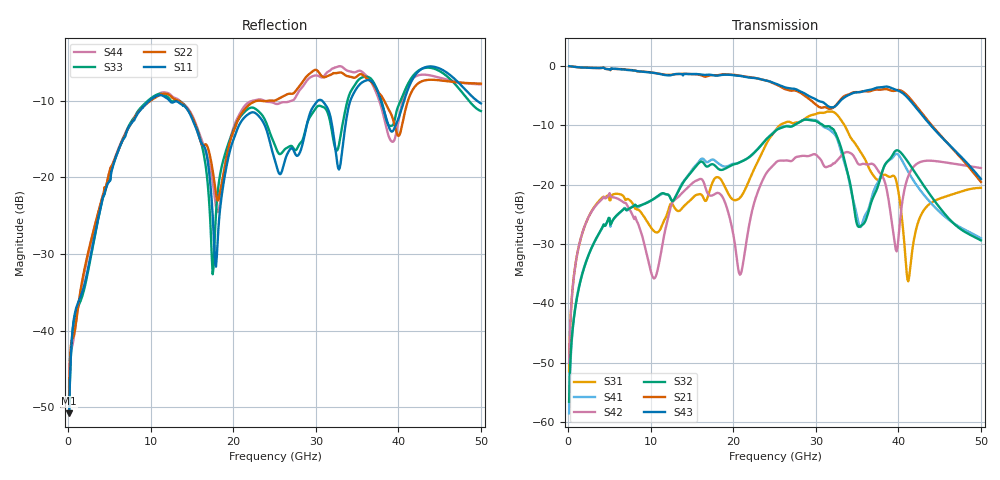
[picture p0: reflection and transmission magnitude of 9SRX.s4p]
! DAC39RF10ACK
! 256-pin FCBGA package
! Texas Instruments 8/20/2022
! Single-ended  S-parameters
! PORT#  PORT_NAME  NET_NAME
! PORT1:  xSRXN.DIEBUMP  xSRXN
! PORT2:  xSRXN.BGA  xSRXN
! PORT3:  xSRXP.DIEBUMP  xSRXP
! PORT4:  xSRXP.BGA  xSRXP
! Touchstone Ver. 1.0
! Number of ports is 4
# Hz	S	MA	R	50.000000
! SCATTERING PARAMETERS  :
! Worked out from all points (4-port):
!   500 points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, 100 MHz to 50 GHz, reference 50 ohm
!   strongest paths, dB at 100 MHz, 12.6 GHz, 25.1 GHz, 37.6 GHz, 50 GHz:
!     S43: 0.0, -1.5, -3.0, -3.6, -19.0
!     S21: 0.0, -1.4, -3.1, -4.0, -19.5
!     S32: -56.5, -22.8, -10.9, -19.9, -29.4
!     S42: -50.0, -23.0, -16.3, -17.7, -17.2
!     S41: -58.5, -22.7, -10.9, -19.4, -29.0
!     S31: -51.4, -23.2, -10.8, -19.2, -20.5
!   lowest |S11| = -50.8 dB at 100 MHz (marker M1), VSWR 1.01, Z = 50.3 + j0.118 ohm
!   |S11| at or under -10 dB: start of sweep to 9.858 GHz; 12.25 GHz to 30.28 GHz (18.03 GHz wide, 84.8 % of centre); 30.73 GHz to 34.19 GHz (3.466 GHz wide, 10.7 % of centre)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
1e8  0.002893 23.9  0.9956 -2.0  0.002735 85.0  0.001494 -103.2
     0.9972 -1.9  0.003786 27.6  0.00121 -97.3  0.003192 80.6
     0.002695 85.2  0.001489 -101.2  0.002919 23.5  0.9942 -2.1
     0.001189 -97.1  0.003158 81.4  0.9971 -1.9  0.004297 25.5
4.1e9  0.0703 36.6  0.9574 -70.6  0.07793 12.0  0.04345 -169.7
       0.9636 -70.3  0.07333 -17.8  0.04307 -169.6  0.07594 21.1
       0.07777 12.0  0.04346 -170.4  0.07002 33.8  0.958 -71.2
       0.04311 -169.0  0.07586 21.0  0.9645 -70.9  0.07282 -16.9
1.01e10  0.324 -69.2  0.8782 -171.6  0.04337 -129.0  0.07406 88.0
         0.8825 -171.7  0.3187 -97.5  0.0746 85.4  0.01761 -129.0
         0.0429 -129.5  0.07404 85.7  0.3298 -72.0  0.8752 -173.2
         0.07419 87.5  0.01767 -129.3  0.8796 -173.1  0.3264 -97.8
2.07e10  0.2185 -76.9  0.8328 10.0  0.07716 -176.1  0.1542 -89.0
         0.8306 9.9  0.2454 -96.5  0.1528 -89.9  0.01791 4.3
         0.07642 -176.5  0.1537 -89.8  0.2418 -84.0  0.8258 7.4
         0.1533 -88.6  0.01802 5.5  0.8279 7.3  0.2548 -96.1
2.98e10  0.2942 -88.8  0.4903 -147.0  0.3924 -118.5  0.3509 68.4
         0.4864 -147.2  0.4981 -133.2  0.3479 65.7  0.1792 -149.0
         0.3897 -118.6  0.3467 66.0  0.2726 -94.6  0.5292 -150.1
         0.351 68.4  0.181 -149.2  0.5332 -150.3  0.4589 -129.2
4.12e10  0.3785 -88.9  0.5672 9.4  0.01766 156.7  0.1382 -135.9
         0.5542 10.9  0.3196 -130.7  0.1449 -131.0  0.1175 108.8
         0.01536 157.7  0.1544 -134.0  0.4095 -98.6  0.5383 1.2
         0.1283 -134.1  0.1182 107.7  0.5334 2.5  0.4007 -130.2
5e10  0.3029 -139.6  0.1037 -122.4  0.09485 -13.9  0.02982 113.1
      0.1056 -120.7  0.4073 -163.7  0.04461 102.0  0.1397 22.9
      0.0941 -14.6  0.03402 101.5  0.27 -136.7  0.1134 -127.1
      0.03545 110.2  0.1383 23.2  0.1119 -127.5  0.403 -165.3
